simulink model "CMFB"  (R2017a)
settings: Solver=ode113  StartTime=0.0  StopTime=3  RelTol=1e-4  EnableMultiTasking=on
model workspace: external: MAT-File (data not in the file)
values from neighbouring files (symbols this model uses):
  Button = readtable('i_button.csv')    [CMFBoptimizer.m]
  Button_Stiffness = table(x_displacement,stiffness,activation_p,activation_d,activation_midair,damping)    [CMFBoptimizer.m]
  Finger = readtable('i_finger.csv')    [CMFBoptimizer.m]
  finger_start_height = random('norm',Finger.fstart_height,Finger.fstart_height_std)    [CMFBoptimizer.m]
  Finger_Stiffness = readtable('i_finger_stiffness.csv')    [CMFBoptimizer.m]
  Sensory = readtable('i_sensorynoise.csv')    [CMFBoptimizer.m]
undefined symbols (not defined in the file or in its folder): amplitude_ag, amplitude_an, b_penvel, Circle, circle_rad, Contact_Forces_Lib, deg, Extr_Data_Ring, Finite, Force, k_pen, kg, Law, Line, line_depth, line_length, m, max_out, min_out, N, PD, pen_exp, phasedelay_ag, PL, pulsewidth_ag, pulsewidth_an, PW, s, step_finish, step_start, to, vis_len_cirFx, vis_len_linBx, vis_len_linBz, vis_opc, vis_opc_en, window, X, Y, Z
libraries: nesl_utility x40, sm_lib x36, Contact_Forces_Lib x2, fl_lib x2, powerlib_meascontrol x1
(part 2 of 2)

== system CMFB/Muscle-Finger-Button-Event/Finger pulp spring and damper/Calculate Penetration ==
  x : Inport
  vx : Inport  Port=2
  Abs : Abs  ZeroCross=off
  Constant : Constant  Value=circle_rad+line_depth
  Dead Zone : DeadZone  LowerValue=-inf  UpperValue=0
  Gain2 : Gain  Gain=-1
  Product : Product
  Sign vx : Signum  ZeroCross=off
  Sign x : Signum  ZeroCross=off
  Sum : Sum  Inputs=+-
  Pos Sign : Outport
  Pen : Outport  Port=2
  Pen Vel : Outport  Port=3
  Vel Sign : Outport  Port=4
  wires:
  x/1 -> Sign x/1, Abs/1
  vx/1 -> Product/2, Sign vx/1
  Constant/1 -> Sum/1
  Sum/1 -> Dead Zone/1
  Abs/1 -> Sum/2
  Sign x/1 -> Pos Sign/1, Product/1
  Sign vx/1 -> Vel Sign/1
  Product/1 -> Gain2/1
  Dead Zone/1 -> Pen/1
  Gain2/1 -> Pen Vel/1

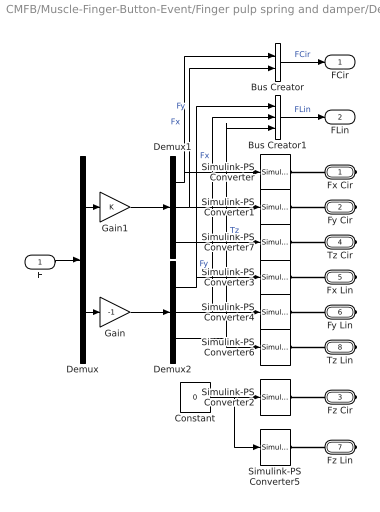
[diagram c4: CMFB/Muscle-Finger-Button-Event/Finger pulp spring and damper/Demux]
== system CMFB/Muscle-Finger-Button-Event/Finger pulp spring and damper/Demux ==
  F : Inport
  Bus Creator : BusCreator  Inputs=2
  Bus Creator1 : BusCreator  Inputs=3
  Constant : Constant  Value=0
  Demux : Demux  Outputs=[3 3]
  Demux1 : Demux  Outputs=3
  Demux2 : Demux  Outputs=3
  Gain : Gain  Gain=-1
  Gain1 : Gain
  Simulink-PS Converter{,1..7} (8 alike) : nesl_utility/Simulink-PS Converter  PhysicalDomain=network_engine_domain  SubClassName=ps_input  LeftPortType=input  RightPortType=output  PseudoPeriodic=off  Frequencies=[]  NoiseDistribution=none  NoiseParameters=[]  Unit=1  AffineConversion=off  FilteringAndDerivatives=zero  SimscapeFilterOrder=1  InputFilterTimeConstant=.001  UdotUserProvided=[]
  Fx Cir : PMIOPort  Port=1  Side=Right
  Fy Cir : PMIOPort  Port=2  Side=Right
  Fz Cir : PMIOPort  Port=3  Side=Right
  Tz Cir : PMIOPort  Port=4  Side=Right
  Fx Lin : PMIOPort  Port=5  Side=Right
  Fy Lin : PMIOPort  Port=6  Side=Right
  Fz Lin : PMIOPort  Port=7  Side=Right
  Tz Lin : PMIOPort  Port=8  Side=Right
  FCir : Outport
  FLin : Outport  Port=2
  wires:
  Bus Creator1/1 -> FLin/1  "FLin"
  Bus Creator/1 -> FCir/1  "FCir"
  Gain1/1 -> Demux1/1
  F/1 -> Demux/1
  Demux/2 -> Gain/1
  Demux/1 -> Gain1/1
  Demux1/1 -> Simulink-PS Converter/1, Bus Creator/1  "Fx"
  Demux1/2 -> Simulink-PS Converter1/1, Bus Creator/2  "Fy"
  Constant/1 -> Simulink-PS Converter2/1, Simulink-PS Converter5/1
  Demux2/2 -> Simulink-PS Converter4/1, Bus Creator1/2  "Fy"
  Demux2/1 -> Simulink-PS Converter3/1, Bus Creator1/1  "Fx"
  Demux2/3 -> Simulink-PS Converter6/1, Bus Creator1/3  "Tz"
  Demux1/3 -> Simulink-PS Converter7/1
  Gain/1 -> Demux2/1
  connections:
  Fz Cir/RConn1 -- Simulink-PS Converter2/RConn1
  Fy Cir/RConn1 -- Simulink-PS Converter1/RConn1
  Fx Cir/RConn1 -- Simulink-PS Converter/RConn1
  Tz Lin/RConn1 -- Simulink-PS Converter6/RConn1
  Fx Lin/RConn1 -- Simulink-PS Converter3/RConn1
  Fy Lin/RConn1 -- Simulink-PS Converter4/RConn1
  Fz Lin/RConn1 -- Simulink-PS Converter5/RConn1
  Tz Cir/RConn1 -- Simulink-PS Converter7/RConn1

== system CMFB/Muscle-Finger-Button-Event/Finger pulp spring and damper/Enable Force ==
  y : Inport
  Abs1 : Abs  ZeroCross=off
  Activation limit for contact force : Constant  Value=line_length/2
  Sum : Sum  Inputs=+-
  Enable : Outport
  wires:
  Abs1/1 -> Sum/2
  y/1 -> Abs1/1
  Activation limit for contact force/1 -> Sum/1
  Sum/1 -> Enable/1

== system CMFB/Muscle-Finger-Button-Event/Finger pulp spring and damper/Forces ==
  M arm : Inport
  X Sep : Inport  Port=2
  Pos Cmp : Inport  Port=3
  Pen : Inport  Port=4
  Vel : Inport  Port=5
  Vel_Cmp : Inport  Port=6
  Unit Vector : Inport  Port=7
  vy : Inport  Port=8
  wz : Inport  Port=9
  Action Port : ActionPort  ActionType=then
  Force Law : Subsystem  AncestorBlock=Contact_Forces_Lib/Force Law  Variant=on  OverrideUsingVariant=Custom
  Mux : Mux  Inputs=6
  Resolve Forces : Subsystem
  Subsystem : Subsystem
  Fnf : Outport  InitialOutput=[0]
  F : Outport  Port=2
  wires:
  Subsystem/1(Out) -> Fnf/1
  Resolve Forces/8(Ff) -> Subsystem/2(Ff)
  Resolve Forces/7(Fn) -> Subsystem/1(Fn)
  Resolve Forces/4(Fx Lin) -> Mux/4
  Pen/1 -> Force Law/1(Pen)
  Vel/1 -> Force Law/2(Pen Vel)
  Resolve Forces/5(Fy Lin) -> Mux/5
  Resolve Forces/6(Tz Lin) -> Mux/6
  Resolve Forces/1(Fx Cir) -> Mux/1
  Resolve Forces/2(Fy Cir) -> Mux/2
  M arm/1 -> Resolve Forces/1(Moment arm)
  Pos Cmp/1 -> Resolve Forces/2(Pos Cmp)
  Mux/1 -> F/1
  Vel_Cmp/1 -> Resolve Forces/6(Vel Cmp)
  Unit Vector/1 -> Resolve Forces/7(Unit Vector)
  wz/1 -> Resolve Forces/9(wz)
  vy/1 -> Resolve Forces/8(vy)
  Resolve Forces/3(Tz Cir) -> Mux/3
  Force Law/1(Spr F) -> Resolve Forces/4(Spr Force Mag)
  Force Law/2(Damp F) -> Resolve Forces/5(Damp Force Mag)
  X Sep/1 -> Resolve Forces/3(X Sep)

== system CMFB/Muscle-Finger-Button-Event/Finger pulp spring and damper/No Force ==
  Action Port : ActionPort  ActionType=else
  Zeros : Constant  Value=[0 0 0 0 0 0]  SampleTime=0
  Zeros1 : Constant  Value=[0 0]  SampleTime=0
  Fnf : Outport  InitialOutput=[0]
  F : Outport  Port=2  InitialOutput=[0 0 0 0 0 0]
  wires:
  Zeros1/1 -> Fnf/1
  Zeros/1 -> F/1

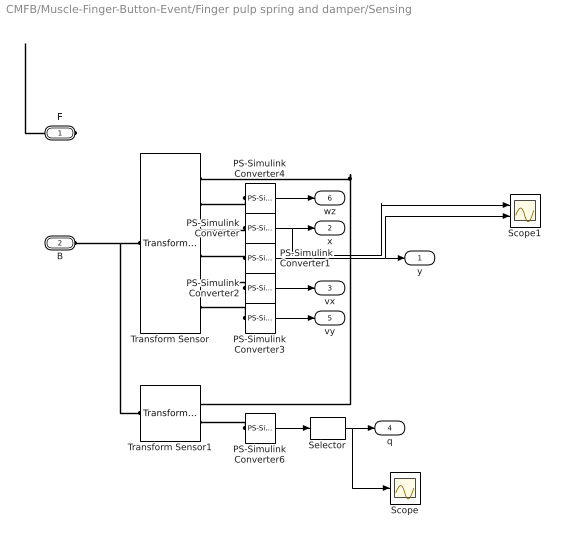
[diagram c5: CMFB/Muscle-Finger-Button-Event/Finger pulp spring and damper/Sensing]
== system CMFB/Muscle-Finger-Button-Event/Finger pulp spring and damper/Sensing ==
  PS-Simulink Converter{,1..4,6} (6 alike) : nesl_utility/PS-Simulink Converter  PhysicalDomain=network_engine_domain  SubClassName=ps_output  LeftPortType=input  RightPortType=output  PseudoPeriodic=off  Frequencies=[]  Unit=1  AffineConversion=off
  Scope : Scope
  Scope1 : Scope  NumInputPorts=2
  Selector : Selector  NumberOfDimensions=2  InputPortWidth=3  IndexOptions=Index vector (dialog),Index vector (dialog)  Indices=[1],[1,2]  OutputSizes=1,1
  Transform Sensor : sm_lib/Frames and Transforms/Transform Sensor  MeasurementFrame=Base  SenseAngle=off  SenseAxis=off  SenseAngle1=off  SenseAngle2=off  SenseAngle3=off  SenseQ=off  SenseR=off  SenseOmegaX=off  SenseOmegaY=off  SenseOmegaZ=on  SenseOmega1=off  SenseOmega2=off  SenseOmega3=off  SenseQDot=off  SenseRDot=off  SenseAlphaX=off  SenseAlphaY=off  SenseAlphaZ=off  SenseAlpha1=off  SenseAlpha2=off  SenseAlpha3=off  SenseQDDot=off  SenseRDDot=off  SenseX=on  SenseY=on  SenseZ=off  SenseRad=off  SenseAzim=off  SenseDist=off  SenseInc=off  SenseXDot=on  SenseYDot=on  SenseZDot=off  SenseRadDot=off  SenseAzimDot=off  SenseDistDot=off  SenseIncDot=off  SenseXDDot=off  SenseYDDot=off  SenseZDDot=off  SenseRadDDot=off  SenseAzimDDot=off  SenseDistDDot=off  SenseIncDDot=off
  Transform Sensor1 : sm_lib/Frames and Transforms/Transform Sensor  MeasurementFrame=World  SenseAngle=off  SenseAxis=off  SenseAngle1=off  SenseAngle2=off  SenseAngle3=off  SenseQ=off  SenseR=on  SenseOmegaX=off  SenseOmegaY=off  SenseOmegaZ=off  SenseOmega1=off  SenseOmega2=off  SenseOmega3=off  SenseQDot=off  SenseRDot=off  SenseAlphaX=off  SenseAlphaY=off  SenseAlphaZ=off  SenseAlpha1=off  SenseAlpha2=off  SenseAlpha3=off  SenseQDDot=off  SenseRDDot=off  SenseX=off  SenseY=off  SenseZ=off  SenseRad=off  SenseAzim=off  SenseDist=off  SenseInc=off  SenseXDot=off  SenseYDot=off  SenseZDot=off  SenseRadDot=off  SenseAzimDot=off  SenseDistDot=off  SenseIncDot=off  SenseXDDot=off  SenseYDDot=off  SenseZDDot=off  SenseRadDDot=off  SenseAzimDDot=off  SenseDistDDot=off  SenseIncDDot=off
  F : PMIOPort  Port=1  Side=Left
  B : PMIOPort  Port=2  Side=Left
  y : Outport
  x : Outport  Port=2
  vx : Outport  Port=3
  q : Outport  Port=4
  vy : Outport  Port=5
  wz : Outport  Port=6
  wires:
  PS-Simulink Converter/1 -> Scope1/1, x/1
  PS-Simulink Converter1/1 -> Scope1/2, y/1
  PS-Simulink Converter2/1 -> vx/1
  PS-Simulink Converter3/1 -> vy/1
  PS-Simulink Converter6/1 -> Selector/1
  Selector/1 -> Scope/1, q/1
  PS-Simulink Converter4/1 -> wz/1
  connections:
  Transform Sensor/RConn1 -- F/RConn1 -- Transform Sensor1/RConn1
  Transform Sensor/LConn1 -- B/RConn1 -- Transform Sensor1/LConn1
  PS-Simulink Converter4/LConn1 -- Transform Sensor/RConn2
  PS-Simulink Converter/LConn1 -- Transform Sensor/RConn3
  PS-Simulink Converter1/LConn1 -- Transform Sensor/RConn4
  PS-Simulink Converter2/LConn1 -- Transform Sensor/RConn5
  PS-Simulink Converter6/LConn1 -- Transform Sensor1/RConn2
  PS-Simulink Converter3/LConn1 -- Transform Sensor/RConn6

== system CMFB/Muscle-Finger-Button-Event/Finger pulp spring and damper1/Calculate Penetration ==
  x : Inport
  vx : Inport  Port=2
  Abs : Abs  ZeroCross=off
  Constant : Constant  Value=circle_rad+line_depth
  Gain2 : Gain  Gain=-1
  Product : Product
  Sign vx : Signum  ZeroCross=off
  Sign x : Signum  ZeroCross=off
  Sum : Sum  Inputs=+-
  Pos Sign : Outport
  Pen : Outport  Port=2
  Pen Vel : Outport  Port=3
  Vel Sign : Outport  Port=4
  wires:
  x/1 -> Sign x/1, Abs/1
  vx/1 -> Product/2, Sign vx/1
  Constant/1 -> Sum/1
  Abs/1 -> Sum/2
  Sign x/1 -> Pos Sign/1, Product/1
  Sign vx/1 -> Vel Sign/1
  Product/1 -> Gain2/1
  Sum/1 -> Pen/1
  Gain2/1 -> Pen Vel/1

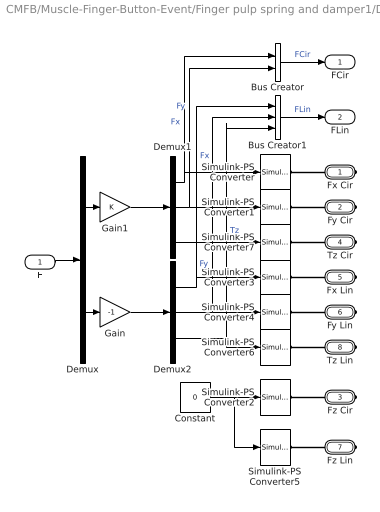
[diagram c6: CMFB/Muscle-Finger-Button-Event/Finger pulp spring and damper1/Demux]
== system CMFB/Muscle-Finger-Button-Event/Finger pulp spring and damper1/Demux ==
  F : Inport
  Bus Creator : BusCreator  Inputs=2
  Bus Creator1 : BusCreator  Inputs=3
  Constant : Constant  Value=0
  Demux : Demux  Outputs=[3 3]
  Demux1 : Demux  Outputs=3
  Demux2 : Demux  Outputs=3
  Gain : Gain  Gain=-1
  Gain1 : Gain
  Simulink-PS Converter{,1..7} (8 alike) : nesl_utility/Simulink-PS Converter  PhysicalDomain=network_engine_domain  SubClassName=ps_input  LeftPortType=input  RightPortType=output  PseudoPeriodic=off  Frequencies=[]  NoiseDistribution=none  NoiseParameters=[]  Unit=1  AffineConversion=off  FilteringAndDerivatives=zero  SimscapeFilterOrder=1  InputFilterTimeConstant=.001  UdotUserProvided=[]
  Fx Cir : PMIOPort  Port=1  Side=Right
  Fy Cir : PMIOPort  Port=2  Side=Right
  Fz Cir : PMIOPort  Port=3  Side=Right
  Tz Cir : PMIOPort  Port=4  Side=Right
  Fx Lin : PMIOPort  Port=5  Side=Right
  Fy Lin : PMIOPort  Port=6  Side=Right
  Fz Lin : PMIOPort  Port=7  Side=Right
  Tz Lin : PMIOPort  Port=8  Side=Right
  FCir : Outport
  FLin : Outport  Port=2
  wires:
  Bus Creator1/1 -> FLin/1  "FLin"
  Bus Creator/1 -> FCir/1  "FCir"
  Gain1/1 -> Demux1/1
  F/1 -> Demux/1
  Demux/2 -> Gain/1
  Demux/1 -> Gain1/1
  Demux1/1 -> Simulink-PS Converter/1, Bus Creator/1  "Fx"
  Demux1/2 -> Simulink-PS Converter1/1, Bus Creator/2  "Fy"
  Constant/1 -> Simulink-PS Converter2/1, Simulink-PS Converter5/1
  Demux2/2 -> Simulink-PS Converter4/1, Bus Creator1/2  "Fy"
  Demux2/1 -> Simulink-PS Converter3/1, Bus Creator1/1  "Fx"
  Demux2/3 -> Simulink-PS Converter6/1, Bus Creator1/3  "Tz"
  Demux1/3 -> Simulink-PS Converter7/1
  Gain/1 -> Demux2/1
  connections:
  Fz Cir/RConn1 -- Simulink-PS Converter2/RConn1
  Fy Cir/RConn1 -- Simulink-PS Converter1/RConn1
  Fx Cir/RConn1 -- Simulink-PS Converter/RConn1
  Tz Lin/RConn1 -- Simulink-PS Converter6/RConn1
  Fx Lin/RConn1 -- Simulink-PS Converter3/RConn1
  Fy Lin/RConn1 -- Simulink-PS Converter4/RConn1
  Fz Lin/RConn1 -- Simulink-PS Converter5/RConn1
  Tz Cir/RConn1 -- Simulink-PS Converter7/RConn1

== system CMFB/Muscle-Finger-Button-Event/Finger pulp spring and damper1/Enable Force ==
  y : Inport
  Abs1 : Abs  ZeroCross=off
  Activation limit for contact force : Constant  Value=line_length/2
  Sum : Sum  Inputs=+-
  Enable : Outport
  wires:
  Abs1/1 -> Sum/2
  y/1 -> Abs1/1
  Activation limit for contact force/1 -> Sum/1
  Sum/1 -> Enable/1

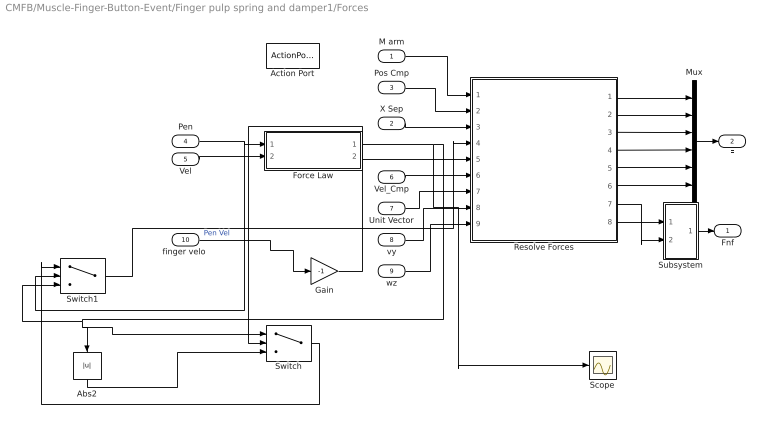
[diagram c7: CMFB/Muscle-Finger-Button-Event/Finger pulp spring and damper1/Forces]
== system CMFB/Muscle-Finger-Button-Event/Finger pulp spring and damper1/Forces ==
  M arm : Inport
  X Sep : Inport  Port=2
  Pos Cmp : Inport  Port=3
  Pen : Inport  Port=4
  Vel : Inport  Port=5
  Vel_Cmp : Inport  Port=6
  Unit Vector : Inport  Port=7
  vy : Inport  Port=8
  wz : Inport  Port=9
  "finger velo " : Inport  Port=10
  Action Port : ActionPort  ActionType=then
  Abs2 : Abs  ZeroCross=off
  Force Law : Subsystem  AncestorBlock=Contact_Forces_Lib/Force Law  Variant=on  OverrideUsingVariant=Custom
  Gain : Gain  Gain=-1
  Mux : Mux  Inputs=6
  Resolve Forces : Subsystem
  Scope : Scope
  Subsystem : Subsystem
  Switch : Switch
  Switch1 : Switch
  Fnf : Outport  InitialOutput=[0]
  F : Outport  Port=2
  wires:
  Subsystem/1(Out) -> Fnf/1
  Resolve Forces/8(Ff) -> Subsystem/2(Ff)
  Resolve Forces/7(Fn) -> Subsystem/1(Fn)
  Resolve Forces/4(Fx Lin) -> Mux/4
  Pen/1 -> Switch1/2, Force Law/1(Pen)
  Vel/1 -> Force Law/2(Pen Vel)
  Resolve Forces/5(Fy Lin) -> Mux/5
  Resolve Forces/6(Tz Lin) -> Mux/6
  Resolve Forces/1(Fx Cir) -> Mux/1
  Resolve Forces/2(Fy Cir) -> Mux/2
  M arm/1 -> Resolve Forces/1(Moment arm)
  Pos Cmp/1 -> Resolve Forces/2(Pos Cmp)
  Mux/1 -> F/1
  Vel_Cmp/1 -> Resolve Forces/6(Vel Cmp)
  Unit Vector/1 -> Resolve Forces/7(Unit Vector)
  wz/1 -> Resolve Forces/9(wz)
  vy/1 -> Resolve Forces/8(vy)
  Resolve Forces/3(Tz Cir) -> Mux/3
  Force Law/2(Damp F) -> Resolve Forces/5(Damp Force Mag)
  X Sep/1 -> Resolve Forces/3(X Sep)
  Abs2/1 -> Switch/3
  "finger velo "/1 -> Gain/1  "Pen Vel"
  Force Law/1(Spr F) -> Switch1/3, Switch/1, Abs2/1, Scope/1
  Gain/1 -> Switch/2
  Switch/1 -> Switch1/1
  Switch1/1 -> Resolve Forces/4(Spr Force Mag)

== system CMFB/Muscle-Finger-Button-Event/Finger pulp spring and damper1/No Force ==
  Action Port : ActionPort  ActionType=else
  Zeros : Constant  Value=[0 0 0 0 0 0]  SampleTime=0
  Zeros1 : Constant  Value=[0 0]  SampleTime=0
  Fnf : Outport  InitialOutput=[0]
  F : Outport  Port=2  InitialOutput=[0 0 0 0 0 0]
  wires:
  Zeros1/1 -> Fnf/1
  Zeros/1 -> F/1

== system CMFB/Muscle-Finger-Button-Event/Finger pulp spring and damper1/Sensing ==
  PS-Simulink Converter{,1..4,6} (6 alike) : nesl_utility/PS-Simulink Converter  PhysicalDomain=network_engine_domain  SubClassName=ps_output  LeftPortType=input  RightPortType=output  PseudoPeriodic=off  Frequencies=[]  Unit=1  AffineConversion=off
  Scope : Scope
  Scope1 : Scope  NumInputPorts=2
  Selector : Selector  NumberOfDimensions=2  InputPortWidth=3  IndexOptions=Index vector (dialog),Index vector (dialog)  Indices=[1],[1,2]  OutputSizes=1,1
  Transform Sensor : sm_lib/Frames and Transforms/Transform Sensor  MeasurementFrame=Base  SenseAngle=off  SenseAxis=off  SenseAngle1=off  SenseAngle2=off  SenseAngle3=off  SenseQ=off  SenseR=off  SenseOmegaX=off  SenseOmegaY=off  SenseOmegaZ=on  SenseOmega1=off  SenseOmega2=off  SenseOmega3=off  SenseQDot=off  SenseRDot=off  SenseAlphaX=off  SenseAlphaY=off  SenseAlphaZ=off  SenseAlpha1=off  SenseAlpha2=off  SenseAlpha3=off  SenseQDDot=off  SenseRDDot=off  SenseX=on  SenseY=on  SenseZ=off  SenseRad=off  SenseAzim=off  SenseDist=off  SenseInc=off  SenseXDot=on  SenseYDot=on  SenseZDot=off  SenseRadDot=off  SenseAzimDot=off  SenseDistDot=off  SenseIncDot=off  SenseXDDot=off  SenseYDDot=off  SenseZDDot=off  SenseRadDDot=off  SenseAzimDDot=off  SenseDistDDot=off  SenseIncDDot=off
  Transform Sensor1 : sm_lib/Frames and Transforms/Transform Sensor  MeasurementFrame=World  SenseAngle=off  SenseAxis=off  SenseAngle1=off  SenseAngle2=off  SenseAngle3=off  SenseQ=off  SenseR=on  SenseOmegaX=off  SenseOmegaY=off  SenseOmegaZ=off  SenseOmega1=off  SenseOmega2=off  SenseOmega3=off  SenseQDot=off  SenseRDot=off  SenseAlphaX=off  SenseAlphaY=off  SenseAlphaZ=off  SenseAlpha1=off  SenseAlpha2=off  SenseAlpha3=off  SenseQDDot=off  SenseRDDot=off  SenseX=off  SenseY=off  SenseZ=off  SenseRad=off  SenseAzim=off  SenseDist=off  SenseInc=off  SenseXDot=off  SenseYDot=off  SenseZDot=off  SenseRadDot=off  SenseAzimDot=off  SenseDistDot=off  SenseIncDot=off  SenseXDDot=off  SenseYDDot=off  SenseZDDot=off  SenseRadDDot=off  SenseAzimDDot=off  SenseDistDDot=off  SenseIncDDot=off
  F : PMIOPort  Port=1  Side=Left
  B : PMIOPort  Port=2  Side=Left
  y : Outport
  x : Outport  Port=2
  vx : Outport  Port=3
  q : Outport  Port=4
  vy : Outport  Port=5
  wz : Outport  Port=6
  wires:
  PS-Simulink Converter/1 -> Scope1/1, x/1
  PS-Simulink Converter1/1 -> Scope1/2, y/1
  PS-Simulink Converter2/1 -> vx/1
  PS-Simulink Converter3/1 -> vy/1
  PS-Simulink Converter6/1 -> Selector/1
  Selector/1 -> Scope/1, q/1
  PS-Simulink Converter4/1 -> wz/1
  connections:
  Transform Sensor/RConn1 -- F/RConn1 -- Transform Sensor1/RConn1
  Transform Sensor/LConn1 -- B/RConn1 -- Transform Sensor1/LConn1
  PS-Simulink Converter4/LConn1 -- Transform Sensor/RConn2
  PS-Simulink Converter/LConn1 -- Transform Sensor/RConn3
  PS-Simulink Converter1/LConn1 -- Transform Sensor/RConn4
  PS-Simulink Converter2/LConn1 -- Transform Sensor/RConn5
  PS-Simulink Converter6/LConn1 -- Transform Sensor1/RConn2
  PS-Simulink Converter3/LConn1 -- Transform Sensor/RConn6

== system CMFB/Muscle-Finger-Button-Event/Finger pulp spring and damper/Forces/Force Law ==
  note: 1) Only subsystems can be added as variant choices at this level 2) Blocks cannot be connected at this level as connectivity is automatically determined at simulation, based on the active variant
  Pen : Inport
  Pen Vel : Inport  Port=2
  Custom : Subsystem  VariantControl=Custom
  Linear : Subsystem  VariantControl=Linear
  Nonlinear : Subsystem  VariantControl=Nonlinear
  Spr F : Outport
  Damp F : Outport  Port=2

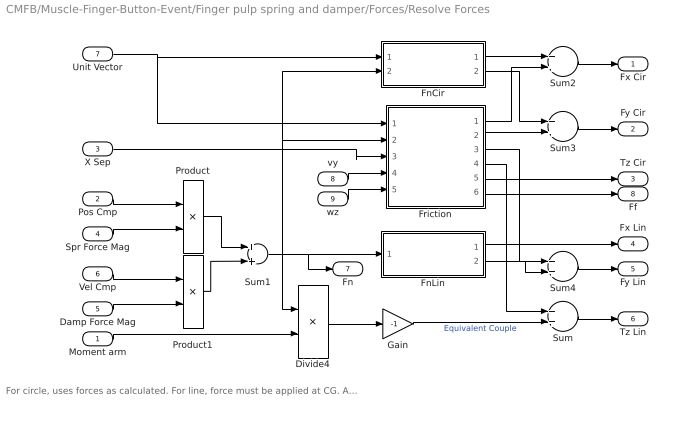
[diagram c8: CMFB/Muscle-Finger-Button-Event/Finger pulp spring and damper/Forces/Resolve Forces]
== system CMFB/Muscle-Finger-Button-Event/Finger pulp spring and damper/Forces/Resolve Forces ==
  note: For circle, uses forces as calculated. For line, force must be applied at CG. Apply torque corresponding to equivalent couple.
  Moment arm : Inport
  Pos Cmp : Inport  Port=2
  X Sep : Inport  Port=3
  Spr Force Mag : Inport  Port=4
  Damp Force Mag : Inport  Port=5
  Vel Cmp : Inport  Port=6
  Unit Vector : Inport  Port=7
  vy : Inport  Port=8
  wz : Inport  Port=9
  Divide4 : Product  Inputs=**
  FnCir : Subsystem
  FnLin : Subsystem
  Friction : Subsystem
  Gain : Gain  Gain=-1
  Product : Product
  Product1 : Product
  Sum{,1..4} (5 alike) : Sum
  Fx Cir : Outport
  Fy Cir : Outport  Port=2
  Tz Cir : Outport  Port=3
  Fx Lin : Outport  Port=4
  Fy Lin : Outport  Port=5
  Tz Lin : Outport  Port=6
  Fn : Outport  Port=7
  Ff : Outport  Port=8
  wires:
  Friction/6(Ff) -> Ff/1
  Product/1 -> Sum1/1
  Spr Force Mag/1 -> Product/2
  Damp Force Mag/1 -> Product1/2
  Product1/1 -> Sum1/2
  Moment arm/1 -> Divide4/2
  Divide4/1 -> Gain/1
  Gain/1 -> Sum/2  "Equivalent Couple"
  Unit Vector/1 -> FnCir/1(Unit Vector), Friction/1(Unit Vector)
  Pos Cmp/1 -> Product/1
  Vel Cmp/1 -> Product1/1
  vy/1 -> Friction/4(vLin)
  wz/1 -> Friction/5(wz)
  Sum/1 -> Tz Lin/1
  Friction/4(TzLin) -> Sum/1
  Friction/1(FxCir) -> Sum2/2
  FnCir/1(FxCir) -> Sum2/1
  FnCir/2(FyCir) -> Sum3/1
  Friction/2(FyCir) -> Sum3/2
  FnLin/2(FyLin) -> Sum4/2
  Friction/3(FyLin) -> Sum4/1
  FnLin/1(FxLin) -> Fx Lin/1
  Sum4/1 -> Fy Lin/1
  Sum3/1 -> Fy Cir/1
  Sum2/1 -> Fx Cir/1
  Sum1/1 -> FnLin/1(Fn), Fn/1, Divide4/1, FnCir/2(Fn), Friction/2(Fn)
  Friction/5(TzCir) -> Tz Cir/1
  X Sep/1 -> Friction/3(X Sep)

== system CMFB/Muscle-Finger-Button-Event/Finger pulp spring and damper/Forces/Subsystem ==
  Fn : Inport
  Ff : Inport  Port=2
  Abs : Abs  ZeroCross=off
  Add : Sum
  Constant : Constant  Value=0
  Mux1 : Mux  Inputs=2
  Out : Outport
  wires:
  Abs/1 -> Mux1/1
  Constant/1 -> Add/2
  Add/1 -> Out/1
  Ff/1 -> Mux1/2
  Fn/1 -> Abs/1
  Mux1/1 -> Add/1

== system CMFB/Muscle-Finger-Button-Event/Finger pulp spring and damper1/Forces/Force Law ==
  note: 1) Only subsystems can be added as variant choices at this level 2) Blocks cannot be connected at this level as connectivity is automatically determined at simulation, based on the active variant
  Pen : Inport
  Pen Vel : Inport  Port=2
  Custom : Subsystem  VariantControl=Custom
  Linear : Subsystem  VariantControl=Linear
  Nonlinear : Subsystem  VariantControl=Nonlinear
  Spr F : Outport
  Damp F : Outport  Port=2

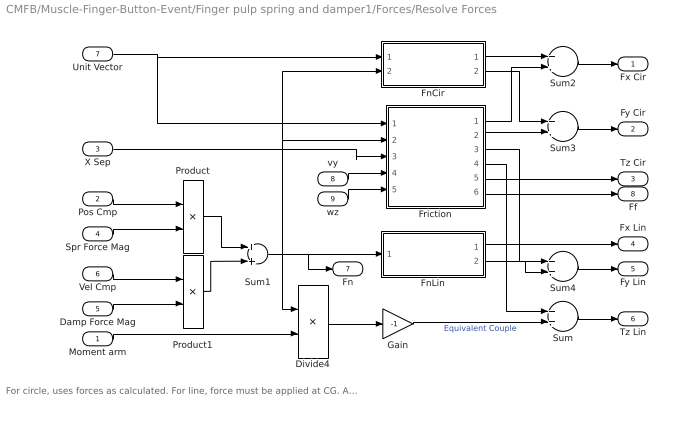
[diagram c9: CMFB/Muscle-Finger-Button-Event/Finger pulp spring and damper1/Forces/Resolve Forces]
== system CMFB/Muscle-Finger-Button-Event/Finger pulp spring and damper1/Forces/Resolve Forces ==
  note: For circle, uses forces as calculated. For line, force must be applied at CG. Apply torque corresponding to equivalent couple.
  Moment arm : Inport
  Pos Cmp : Inport  Port=2
  X Sep : Inport  Port=3
  Spr Force Mag : Inport  Port=4
  Damp Force Mag : Inport  Port=5
  Vel Cmp : Inport  Port=6
  Unit Vector : Inport  Port=7
  vy : Inport  Port=8
  wz : Inport  Port=9
  Divide4 : Product  Inputs=**
  FnCir : Subsystem
  FnLin : Subsystem
  Friction : Subsystem
  Gain : Gain  Gain=-1
  Product : Product
  Product1 : Product
  Sum{,1..4} (5 alike) : Sum
  Fx Cir : Outport
  Fy Cir : Outport  Port=2
  Tz Cir : Outport  Port=3
  Fx Lin : Outport  Port=4
  Fy Lin : Outport  Port=5
  Tz Lin : Outport  Port=6
  Fn : Outport  Port=7
  Ff : Outport  Port=8
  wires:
  Friction/6(Ff) -> Ff/1
  Product/1 -> Sum1/1
  Spr Force Mag/1 -> Product/2
  Damp Force Mag/1 -> Product1/2
  Product1/1 -> Sum1/2
  Moment arm/1 -> Divide4/2
  Divide4/1 -> Gain/1
  Gain/1 -> Sum/2  "Equivalent Couple"
  Unit Vector/1 -> FnCir/1(Unit Vector), Friction/1(Unit Vector)
  Pos Cmp/1 -> Product/1
  Vel Cmp/1 -> Product1/1
  vy/1 -> Friction/4(vLin)
  wz/1 -> Friction/5(wz)
  Sum/1 -> Tz Lin/1
  Friction/4(TzLin) -> Sum/1
  Friction/1(FxCir) -> Sum2/2
  FnCir/1(FxCir) -> Sum2/1
  FnCir/2(FyCir) -> Sum3/1
  Friction/2(FyCir) -> Sum3/2
  FnLin/2(FyLin) -> Sum4/2
  Friction/3(FyLin) -> Sum4/1
  FnLin/1(FxLin) -> Fx Lin/1
  Sum4/1 -> Fy Lin/1
  Sum3/1 -> Fy Cir/1
  Sum2/1 -> Fx Cir/1
  Sum1/1 -> FnLin/1(Fn), Fn/1, Divide4/1, FnCir/2(Fn), Friction/2(Fn)
  Friction/5(TzCir) -> Tz Cir/1
  X Sep/1 -> Friction/3(X Sep)

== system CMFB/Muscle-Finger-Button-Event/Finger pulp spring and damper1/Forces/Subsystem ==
  Fn : Inport
  Ff : Inport  Port=2
  Abs : Abs  ZeroCross=off
  Add : Sum
  Constant : Constant  Value=0
  Mux1 : Mux  Inputs=2
  Out : Outport
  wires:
  Abs/1 -> Mux1/1
  Constant/1 -> Add/2
  Add/1 -> Out/1
  Ff/1 -> Mux1/2
  Fn/1 -> Abs/1
  Mux1/1 -> Add/1

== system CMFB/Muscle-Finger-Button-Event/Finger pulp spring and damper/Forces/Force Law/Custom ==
  note: Implement your own custom force law in this subsystem. To use it in the contact force models, set the parameter "Force Law" to "Custom".
  Pen : Inport
  Pen Vel : Inport  Port=2
  1-D Lookup Table : Lookup_n-D  NumberOfTableDimensions=1  BreakpointsForDimension1=Finger_Stiffness.displacement  Table=Finger_Stiffness.stiffness  InternalRulePriority=Speed  RndMeth=Simplest
  Abs : Abs  ZeroCross=off
  Abs1 : Abs  ZeroCross=off
  Gain2 : Gain  Gain=-1.5  Multiplication=Matrix(K*u)
  Product : Product
  Product1 : Product
  Saturation : Saturate  UpperLimit=Inf  LowerLimit=0  ZeroCross=off
  Sign : Signum  ZeroCross=off
  Spr F : Outport
  Damp F : Outport  Port=2
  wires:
  Saturation/1 -> Gain2/1
  Pen/1 -> Sign/1, Abs1/1  "Penetration"
  Abs/1 -> Product/1  "Damping_Force_Enable"
  Product/1 -> Damp F/1  "Damping_Force"
  Sign/1 -> Abs/1
  Pen Vel/1 -> Saturation/1  "Pen Vel"
  Gain2/1 -> Product/2  "Damping_Force"
  1-D Lookup Table/1 -> Product1/2
  Abs1/1 -> Product1/1, 1-D Lookup Table/1
  Product1/1 -> Spr F/1

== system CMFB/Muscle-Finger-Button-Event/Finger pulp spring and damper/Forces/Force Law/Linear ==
  Pen : Inport
  Pen Vel : Inport  Port=2
  Abs : Abs  ZeroCross=off
  Gain1 : Gain  Gain=k_pen  Multiplication=Matrix(K*u)
  Gain2 : Gain  Gain=-b_penvel  Multiplication=Matrix(K*u)
  Product : Product
  Saturation : Saturate  UpperLimit=Inf  LowerLimit=0  ZeroCross=off
  Sign : Signum  ZeroCross=off
  Spr F : Outport
  Damp F : Outport  Port=2
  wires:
  Saturation/1 -> Gain2/1
  Pen/1 -> Sign/1, Gain1/1  "Penetration"
  Abs/1 -> Product/1  "Damping_Force_Enable"
  Product/1 -> Damp F/1  "Damping_Force"
  Sign/1 -> Abs/1
  Pen Vel/1 -> Saturation/1  "Pen Vel"
  Gain2/1 -> Product/2  "Damping_Force"
  Gain1/1 -> Spr F/1  "Stiffness_Force"

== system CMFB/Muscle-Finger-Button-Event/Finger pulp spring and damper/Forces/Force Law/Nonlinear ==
  Pen : Inport
  Pen Vel : Inport  Port=2
  Constant : Constant  Value=pen_exp
  Gain1 : Gain  Gain=k_pen  Multiplication=Matrix(K*u)
  Gain2 : Gain  Gain=-b_penvel  Multiplication=Matrix(K*u)
  Math Function : Math  Operator=pow
  Product1 : Product
  Saturation : Saturate  UpperLimit=Inf  LowerLimit=0  ZeroCross=off
  Smoothstep : Subsystem
  Spr F : Outport
  Damp F : Outport  Port=2
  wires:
  Saturation/1 -> Gain2/1
  Product1/1 -> Damp F/1
  Smoothstep/1(Out1) -> Product1/1  "Damping_Enable"
  Gain2/1 -> Product1/2  "Damping_Force"
  Constant/1 -> Math Function/2
  Math Function/1 -> Gain1/1
  Pen/1 -> Math Function/1, Smoothstep/1(In1)  "Penetration"
  Pen Vel/1 -> Saturation/1  "Penetration_Velocity"
  Gain1/1 -> Spr F/1  "Stiffness_Force"

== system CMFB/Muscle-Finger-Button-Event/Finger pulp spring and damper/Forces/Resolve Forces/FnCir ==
  note: Calculate circle Normal Force in circle reference frame
  Unit Vector : Inport
  Fn : Inport  Port=2
  Demux1 : Demux  Outputs=2
  Divide1 : Product  Inputs=**
  FxCir : Outport
  FyCir : Outport  Port=2
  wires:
  Demux1/1 -> FxCir/1  "Fx Cir"
  Demux1/2 -> FyCir/1  "Fy Cir"
  Fn/1 -> Divide1/1
  Divide1/1 -> Demux1/1
  Unit Vector/1 -> Divide1/2

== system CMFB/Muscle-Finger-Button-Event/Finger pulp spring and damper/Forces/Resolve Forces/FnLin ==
  note: Normal Force is calculated in line reference frame, and acts along x-axis only.
  Fn : Inport
  Constant : Constant  Value=0
  Constant1 : Constant  Value=0
  Sum : Sum
  FxLin : Outport
  FyLin : Outport  Port=2
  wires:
  Constant/1 -> FyLin/1  "Fy Lin"
  Fn/1 -> Sum/2  "Fx Lin"
  Sum/1 -> FxLin/1
  Constant1/1 -> Sum/1

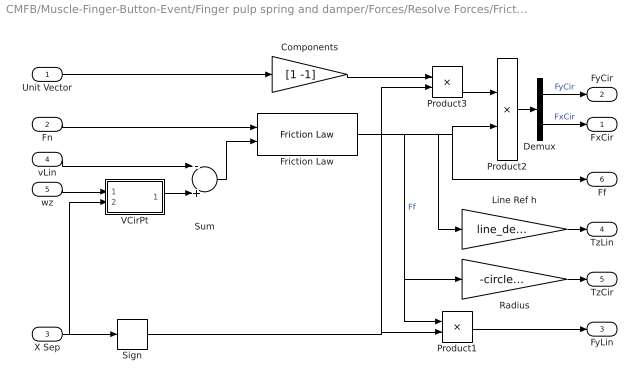
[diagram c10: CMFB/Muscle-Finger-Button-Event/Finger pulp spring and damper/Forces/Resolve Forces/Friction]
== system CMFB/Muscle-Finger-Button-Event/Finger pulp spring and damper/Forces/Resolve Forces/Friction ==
  Unit Vector : Inport
  Fn : Inport  Port=2
  X Sep : Inport  Port=3
  vLin : Inport  Port=4
  wz : Inport  Port=5
  Components : Gain  Gain=[1 -1]
  Demux : Demux  Outputs=2
  Friction Law : Contact_Forces_Lib/Friction Law  OverrideUsingVariant=None
  Line Ref h : Gain  Gain=line_depth
  Product1 : Product
  Product2 : Product
  Product3 : Product
  Radius : Gain  Gain=-circle_rad
  Sign : Signum
  Sum : Sum  Inputs=-+
  VCirPt : Subsystem
  FxCir : Outport
  FyCir : Outport  Port=2
  FyLin : Outport  Port=3
  TzLin : Outport  Port=4
  TzCir : Outport  Port=5
  Ff : Outport  Port=6
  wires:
  Product3/1 -> Product2/1
  Components/1 -> Product3/1
  Product1/1 -> FyLin/1
  Friction Law/1 -> Line Ref h/1, Product2/2, Ff/1, Radius/1, Product1/1  "Ff"
  Demux/1 -> FyCir/1  "FyCir"
  vLin/1 -> Sum/1
  VCirPt/1(vCir) -> Sum/2
  Demux/2 -> FxCir/1  "FxCir"
  wz/1 -> VCirPt/1(wz)
  Unit Vector/1 -> Components/1
  Sum/1 -> Friction Law/2
  Fn/1 -> Friction Law/1
  Line Ref h/1 -> TzLin/1
  Radius/1 -> TzCir/1
  Product2/1 -> Demux/1
  X Sep/1 -> Sign/1, VCirPt/2(X sep)
  Sign/1 -> Product1/2, Product3/2

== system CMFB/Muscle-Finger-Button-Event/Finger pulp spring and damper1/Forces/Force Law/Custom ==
  note: Implement your own custom force law in this subsystem. To use it in the contact force models, set the parameter "Force Law" to "Custom".
  Pen : Inport
  Pen Vel : Inport  Port=2
  1-D Lookup Table : Lookup_n-D  NumberOfTableDimensions=1  BreakpointsForDimension1=Button_Stiffness.x_displacement  Table=Button_Stiffness.stiffness  InternalRulePriority=Speed  RndMeth=Simplest
  Abs : Abs  ZeroCross=off
  Abs1 : Abs  ZeroCross=off
  Constant : Constant  Value=0
  Gain1 : Gain  Gain=k_pen  Multiplication=Matrix(K*u)
  Gain2 : Gain  Gain=0  Multiplication=Matrix(K*u)
  Product : Product
  Product1 : Product
  Saturation : Saturate  UpperLimit=Inf  LowerLimit=0  ZeroCross=off
  Scope : Scope
  Scope1 : Scope
  Sign : Signum  ZeroCross=off
  Spr F : Outport
  Damp F : Outport  Port=2
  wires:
  Saturation/1 -> Gain2/1
  Pen/1 -> Abs1/1, Product1/1, Sign/1, Gain1/1  "Penetration"
  Product/1 -> Damp F/1  "Damping_Force"
  Sign/1 -> Abs/1
  Pen Vel/1 -> Scope1/1, Saturation/1  "Pen Vel"
  Gain2/1 -> Product/2  "Damping_Force"
  Product1/1 -> Spr F/1  "stiffness force"
  Abs1/1 -> Scope/1, 1-D Lookup Table/1
  Constant/1 -> Product/1
  1-D Lookup Table/1 -> Product1/2

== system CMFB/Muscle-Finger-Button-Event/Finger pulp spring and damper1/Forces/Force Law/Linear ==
  Pen : Inport
  Pen Vel : Inport  Port=2
  Abs : Abs  ZeroCross=off
  Gain1 : Gain  Gain=k_pen  Multiplication=Matrix(K*u)
  Gain2 : Gain  Gain=-b_penvel  Multiplication=Matrix(K*u)
  Product : Product
  Saturation : Saturate  UpperLimit=Inf  LowerLimit=0  ZeroCross=off
  Sign : Signum  ZeroCross=off
  Spr F : Outport
  Damp F : Outport  Port=2
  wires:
  Saturation/1 -> Gain2/1
  Pen/1 -> Sign/1, Gain1/1  "Penetration"
  Abs/1 -> Product/1  "Damping_Force_Enable"
  Product/1 -> Damp F/1  "Damping_Force"
  Sign/1 -> Abs/1
  Pen Vel/1 -> Saturation/1  "Pen Vel"
  Gain2/1 -> Product/2  "Damping_Force"
  Gain1/1 -> Spr F/1  "Stiffness_Force"

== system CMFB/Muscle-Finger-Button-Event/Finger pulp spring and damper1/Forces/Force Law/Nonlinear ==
  Pen : Inport
  Pen Vel : Inport  Port=2
  Constant : Constant  Value=pen_exp
  Gain1 : Gain  Gain=k_pen  Multiplication=Matrix(K*u)
  Gain2 : Gain  Gain=-b_penvel  Multiplication=Matrix(K*u)
  Math Function : Math  Operator=pow
  Product1 : Product
  Saturation : Saturate  UpperLimit=Inf  LowerLimit=0  ZeroCross=off
  Smoothstep : Subsystem
  Spr F : Outport
  Damp F : Outport  Port=2
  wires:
  Saturation/1 -> Gain2/1
  Product1/1 -> Damp F/1
  Smoothstep/1(Out1) -> Product1/1  "Damping_Enable"
  Gain2/1 -> Product1/2  "Damping_Force"
  Constant/1 -> Math Function/2
  Math Function/1 -> Gain1/1
  Pen/1 -> Math Function/1, Smoothstep/1(In1)  "Penetration"
  Pen Vel/1 -> Saturation/1  "Penetration_Velocity"
  Gain1/1 -> Spr F/1  "Stiffness_Force"

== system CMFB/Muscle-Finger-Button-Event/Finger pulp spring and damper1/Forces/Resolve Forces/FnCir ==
  note: Calculate circle Normal Force in circle reference frame
  Unit Vector : Inport
  Fn : Inport  Port=2
  Demux1 : Demux  Outputs=2
  Divide1 : Product  Inputs=**
  FxCir : Outport
  FyCir : Outport  Port=2
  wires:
  Demux1/1 -> FxCir/1  "Fx Cir"
  Demux1/2 -> FyCir/1  "Fy Cir"
  Fn/1 -> Divide1/1
  Divide1/1 -> Demux1/1
  Unit Vector/1 -> Divide1/2

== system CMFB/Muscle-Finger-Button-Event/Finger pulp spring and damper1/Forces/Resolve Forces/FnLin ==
  note: Normal Force is calculated in line reference frame, and acts along x-axis only.
  Fn : Inport
  Constant : Constant  Value=0
  Constant1 : Constant  Value=0
  Sum : Sum
  FxLin : Outport
  FyLin : Outport  Port=2
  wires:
  Constant/1 -> FyLin/1  "Fy Lin"
  Fn/1 -> Sum/2  "Fx Lin"
  Sum/1 -> FxLin/1
  Constant1/1 -> Sum/1

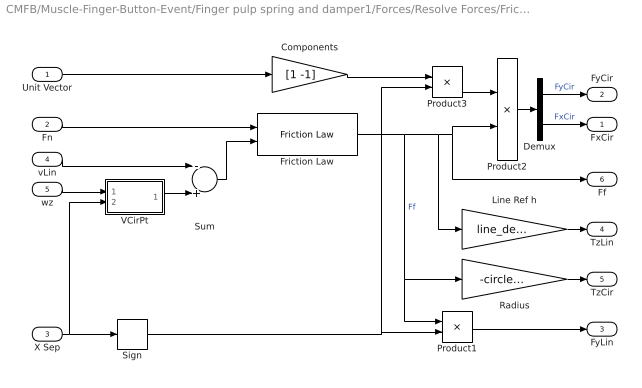
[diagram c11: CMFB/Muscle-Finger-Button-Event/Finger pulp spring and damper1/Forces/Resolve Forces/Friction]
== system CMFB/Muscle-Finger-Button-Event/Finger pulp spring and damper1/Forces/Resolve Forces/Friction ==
  Unit Vector : Inport
  Fn : Inport  Port=2
  X Sep : Inport  Port=3
  vLin : Inport  Port=4
  wz : Inport  Port=5
  Components : Gain  Gain=[1 -1]
  Demux : Demux  Outputs=2
  Friction Law : Contact_Forces_Lib/Friction Law  OverrideUsingVariant=None
  Line Ref h : Gain  Gain=line_depth
  Product1 : Product
  Product2 : Product
  Product3 : Product
  Radius : Gain  Gain=-circle_rad
  Sign : Signum
  Sum : Sum  Inputs=-+
  VCirPt : Subsystem
  FxCir : Outport
  FyCir : Outport  Port=2
  FyLin : Outport  Port=3
  TzLin : Outport  Port=4
  TzCir : Outport  Port=5
  Ff : Outport  Port=6
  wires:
  Product3/1 -> Product2/1
  Components/1 -> Product3/1
  Product1/1 -> FyLin/1
  Friction Law/1 -> Line Ref h/1, Product2/2, Ff/1, Radius/1, Product1/1  "Ff"
  Demux/1 -> FyCir/1  "FyCir"
  vLin/1 -> Sum/1
  VCirPt/1(vCir) -> Sum/2
  Demux/2 -> FxCir/1  "FxCir"
  wz/1 -> VCirPt/1(wz)
  Unit Vector/1 -> Components/1
  Sum/1 -> Friction Law/2
  Fn/1 -> Friction Law/1
  Line Ref h/1 -> TzLin/1
  Radius/1 -> TzCir/1
  Product2/1 -> Demux/1
  X Sep/1 -> Sign/1, VCirPt/2(X sep)
  Sign/1 -> Product1/2, Product3/2

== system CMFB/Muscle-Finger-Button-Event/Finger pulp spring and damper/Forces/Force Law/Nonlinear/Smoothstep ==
  In1 : Inport
  Clamp : Saturate  UpperLimit=step_finish  LowerLimit=step_start
  Constant : Constant  Value=3
  Divide : Product  Inputs=*/
  Divide1 : Product  Inputs=****
  Gain : Gain  Gain=2
  Subtract : Sum  Inputs=+-
  Subtract1 : Sum  Inputs=-+
  Subtract2 : Sum
  Subtract3 : Sum  Inputs=+-
  Subtract4 : Sum  Inputs=+-
  max out : Constant  Value=max_out
  min out : Constant  Value=min_out
  step finish : Constant  Value=step_finish
  step start : Constant  Value=step_start
  Out1 : Outport
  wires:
  step start/1 -> Subtract1/1, Subtract/2
  In1/1 -> Clamp/1
  Subtract1/1 -> Divide/2
  Divide/1 -> Gain/1, Divide1/2, Divide1/3
  Subtract/1 -> Divide/1
  Subtract2/1 -> Out1/1
  Constant/1 -> Subtract4/1
  min out/1 -> Subtract2/2, Subtract3/2
  max out/1 -> Subtract3/1
  Clamp/1 -> Subtract/1
  step finish/1 -> Subtract1/2
  Divide1/1 -> Subtract2/1
  Gain/1 -> Subtract4/2
  Subtract4/1 -> Divide1/1
  Subtract3/1 -> Divide1/4

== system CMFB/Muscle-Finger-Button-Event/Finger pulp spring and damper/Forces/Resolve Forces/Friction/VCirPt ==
  wz : Inport
  X sep : Inport  Port=2
  Constant : Constant  Value=line_depth
  Product : Product
  Product1 : Product
  Sign1 : Signum
  Subtract : Sum  Inputs=+-
  vCir : Outport
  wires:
  Subtract/1 -> Product1/2
  Constant/1 -> Product/2
  X sep/1 -> Sign1/1, Subtract/1
  Sign1/1 -> Product/1
  Product/1 -> Subtract/2
  Product1/1 -> vCir/1
  wz/1 -> Product1/1

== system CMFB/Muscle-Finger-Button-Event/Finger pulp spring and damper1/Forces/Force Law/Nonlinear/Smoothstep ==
  In1 : Inport
  Clamp : Saturate  UpperLimit=step_finish  LowerLimit=step_start
  Constant : Constant  Value=3
  Divide : Product  Inputs=*/
  Divide1 : Product  Inputs=****
  Gain : Gain  Gain=2
  Subtract : Sum  Inputs=+-
  Subtract1 : Sum  Inputs=-+
  Subtract2 : Sum
  Subtract3 : Sum  Inputs=+-
  Subtract4 : Sum  Inputs=+-
  max out : Constant  Value=max_out
  min out : Constant  Value=min_out
  step finish : Constant  Value=step_finish
  step start : Constant  Value=step_start
  Out1 : Outport
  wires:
  step start/1 -> Subtract1/1, Subtract/2
  In1/1 -> Clamp/1
  Subtract1/1 -> Divide/2
  Divide/1 -> Gain/1, Divide1/2, Divide1/3
  Subtract/1 -> Divide/1
  Subtract2/1 -> Out1/1
  Constant/1 -> Subtract4/1
  min out/1 -> Subtract2/2, Subtract3/2
  max out/1 -> Subtract3/1
  Clamp/1 -> Subtract/1
  step finish/1 -> Subtract1/2
  Divide1/1 -> Subtract2/1
  Gain/1 -> Subtract4/2
  Subtract4/1 -> Divide1/1
  Subtract3/1 -> Divide1/4

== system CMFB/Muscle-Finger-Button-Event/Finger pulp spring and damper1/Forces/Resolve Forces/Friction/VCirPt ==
  wz : Inport
  X sep : Inport  Port=2
  Constant : Constant  Value=line_depth
  Product : Product
  Product1 : Product
  Sign1 : Signum
  Subtract : Sum  Inputs=+-
  vCir : Outport
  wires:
  Subtract/1 -> Product1/2
  Constant/1 -> Product/2
  X sep/1 -> Sign1/1, Subtract/1
  Sign1/1 -> Product/1
  Product/1 -> Subtract/2
  Product1/1 -> vCir/1
  wz/1 -> Product1/1
